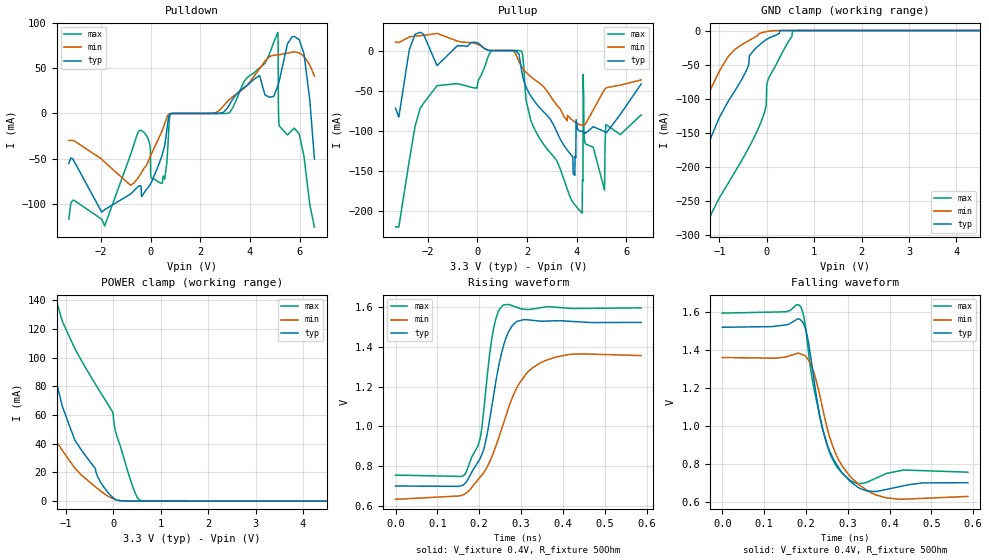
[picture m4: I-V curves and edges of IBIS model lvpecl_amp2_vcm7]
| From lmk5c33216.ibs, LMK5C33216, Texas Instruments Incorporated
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[Model]   lvpecl_amp2_vcm7
Model_type   Output
Polarity   Non-Inverting
Vmeas = 1.1
Vref = 0.4
Cref = 0pF
Rref = 50
|   typ   min   max
C_comp   0.65pF   0.575pF   0.725pF
[Voltage Range]   3.3   3.135   3.465
[Temperature Range]   50   135   -40
[Pullup Reference]   3.3   3.135   3.465
[Pulldown Reference]   0   0   0
[Power Clamp Reference]   3.3   3.135   3.465
[GND Clamp Reference]   0   0   0
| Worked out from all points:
|   slope of the pulldown table from 0 to 0.495 V, typ, clamps not added: 14.2 ohm
|   slope of the pullup table from 0 to 0.495 V, typ, clamps not added: 51.8 ohm
|   falling waveform, V_fixture 0.4V, R_fixture 50Ohm: 20-80 % time 45.2ps typ, 64ps min, 43.1ps max; typ from 1.52 V to 0.7 V
|   rising waveform, V_fixture 0.4V, R_fixture 50Ohm: 20-80 % time 44.9ps typ, 80.5ps min, 29.3ps max; typ from 0.7 V to 1.52 V
[Pulldown]
|   Voltage   I(typ)   I(min)   I(max)
-3.3V     -55.39mA   -29.91mA   -116.7mA
-1.855V   -106.3mA   -53.89mA   -124.3mA
-815.1mV  -89.11mA   -79.31mA   -45.88mA
-280.5mV  -88.39mA   -61.13mA   -20.78mA
462mV     -46.15mA   -18.92mA   -77.03mA
798.6mV   -286.9uA   -140.5uA   -475.4uA
3.155V    8.846mA    14.92mA    609.3uA
5.125V    30.42mA    64.69mA    89.66mA
5.145V    32.3mA     64.75mA    14.89mA
5.174V    35.37mA    64.86mA    -12.6mA
5.986V    81.56mA    67mA       -22.65mA
6.6V      -50.44mA   41.43mA    -125.7mA
[GND Clamp]
|   Voltage   I(typ)   I(min)   I(max)
-3.3V     -892.9mA   -765.6mA   -1.068A
-1.924V   -314.6mA   -288.5mA   -459.9mA
-1.815V   -287mA     -251.4mA   -425.6mA
-1.478V   -218.2mA   -143.5mA   -333.1mA
-1.162V   -154.3mA   -82.94mA   -268mA
-815.1mV  -104mA     -38.12mA   -224.4mA
-171.6mV  -22.09mA   -4.573mA   -142.5mA
-13.2mV   -13.46mA   -1.685mA   -109.6mA
-3.3mV    -13.01mA   -1.546mA   -81.32mA
26.4mV    -11.77mA   -1.169mA   -72.35mA
551.1mV   0A         -83.65nA   -742.2uA
6.6V      0A         0A         0A
[Pullup]
|   Voltage   I(typ)   I(min)   I(max)
-3.3V     -71.72mA   10.75mA    -218.9mA
-2.3V     22.63mA    18.42mA    -71.41mA
570.9mV   -32.22uA   35.11uA    -439.1uA
1.789V    -26.17mA   -20.57mA   -1.239mA
3.858V    -153.3mA   -87.23mA   -189mA
4.224V    -100.2mA   -92.52mA   -202.1mA
4.254V    -100.4mA   -92.42mA   -162.3mA
4.264V    -100.6mA   -92.38mA   -29.77mA
4.333V    -102.7mA   -92.05mA   -114.8mA
5.125V    -100.8mA   -48.16mA   -173.6mA
5.174V    -102.1mA   -46.94mA   -92.62mA
6.6V      -41.63mA   -36.46mA   -80.01mA
[POWER Clamp]
|   Voltage   I(typ)   I(min)   I(max)
-3.3V     330.7mA    180mA      566.4mA
-2.736V   200mA      135.8mA    401.6mA
-1.647V   138.3mA    65.17mA    197.7mA
-1.459V   117.6mA    55.06mA    168.7mA
-1.082V   66.76mA    35.64mA    126mA
-815.1mV  42.67mA    23.06mA    106.5mA
-3.3mV    2.23mA     1.644mA    59.85mA
46.2mV    1.16mA     1.045mA    48.48mA
313.5mV   86.42uA    94.45uA    19.62mA
491.7mV   74.41uA    72.76uA    3.272mA
570.9mV   69.96uA    68.47uA    464.4uA
6.6V      0A         0A         0A
[Ramp]
R_load = 50
|   typ   min   max
dV/dt_r   0.493222/4.44764e-11   0.433502/8.0457e-11   0.504255/2.88608e-11
dV/dt_f   0.492758/4.51803e-11   0.440388/6.34859e-11   0.504255/4.30426e-11
[Falling Waveform]
V_fixture = 0.4V
V_fixture_min = 0.35V
V_fixture_max = 0.45V
R_fixture = 50Ohm
C_fixture = 0F
|   Time   V(typ)   V(min)   V(max)
0s        1.521V     1.361V     1.596V
185.2ps   1.563V     1.381V     1.636V
197ps     1.526V     1.372V     1.552V
213.2ps   1.338V     1.316V     1.274V
232.6ps   1.06V      1.167V     1.054V
248.2ps   921.3mV    1.012V     915.9mV
272.9ps   798.1mV    843.8mV    786.7mV
305ps     708.1mV    735.1mV    713.4mV
389.7ps   662.7mV    620.4mV    745.6mV
587.2ps   699.5mV    626.9mV    755.1mV
[Rising Waveform]
V_fixture = 0.4V
V_fixture_min = 0.35V
V_fixture_max = 0.45V
R_fixture = 50Ohm
C_fixture = 0F
|   Time   V(typ)   V(min)   V(max)
0s        700.4mV    633.3mV    755.1mV
167ps     716mV      662.5mV    763mV
201.6ps   835.5mV    743.2mV    934mV
211.3ps   887.9mV    768.8mV    1.087V
232.9ps   1.135V     861.1mV    1.475V
244.5ps   1.28V      928.9mV    1.57V
257ps     1.396V     1.008V     1.609V
287.5ps   1.523V     1.182V     1.6V
349.4ps   1.529V     1.322V     1.597V
587.2ps   1.522V     1.356V     1.596V
